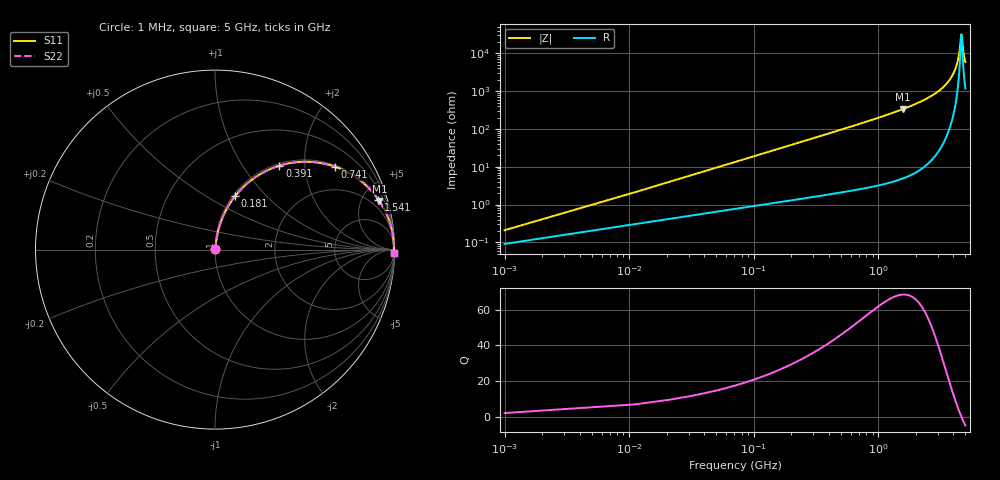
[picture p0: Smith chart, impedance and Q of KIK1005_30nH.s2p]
!version-3
!date-01.2023
!Series
# MHz S RI R 50
!Freq ReS11 ImS11 ReS21 ImS21 ReS12 ImS12 ReS22 ImS22
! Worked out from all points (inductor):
!   501 points, 1 MHz to 5 GHz, reference 50 ohm
!   read as one part in series: L = 30 nH near 21 MHz
!   highest Q = 68.5 at 1.581 GHz (marker M1), where L = 33.9 nH
!   self-resonance near 4.641 GHz
!   S11 on the Smith chart (normalised r, x): 1 MHz: 1.00, +0.00; 181 MHz: 1.02, +0.68; 391 MHz: 1.04, +1.48; 741 MHz: 1.05, +2.87; 1.541 GHz: 1.10, +6.53; 5 GHz: open
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1  0.00091 0.00188  0.9991 -0.00188  0.9991 -0.00188  0.00091 0.00188
31  0.00838 0.0577  0.9916 -0.0577  0.9916 -0.0577  0.00838 0.0577
51  0.0154 0.0941  0.9846 -0.0941  0.9846 -0.0941  0.0154 0.0941
101  0.0431 0.1806  0.9569 -0.1806  0.9569 -0.1806  0.0431 0.1806
181  0.1131 0.2994  0.8869 -0.2994  0.8869 -0.2994  0.1131 0.2994
271  0.215 0.3964  0.785 -0.3964  0.785 -0.3964  0.215 0.3964
391  0.3587 0.4675  0.6413 -0.4675  0.6413 -0.4675  0.3587 0.4675
741  0.6697 0.4613  0.3303 -0.4613  0.3303 -0.4613  0.6697 0.4613
841  0.7253 0.4378  0.2747 -0.4378  0.2747 -0.4378  0.7253 0.4378
1141  0.8359 0.3627  0.1641 -0.3627  0.1641 -0.3627  0.8359 0.3627
1541  0.9108 0.2778  0.0892 -0.2778  0.0892 -0.2778  0.9108 0.2778
1581  0.9158 0.2705  0.0842 -0.2705  0.0842 -0.2705  0.9158 0.2705
1671  0.9258 0.2548  0.0742 -0.2548  0.0742 -0.2548  0.9258 0.2548
2501  0.9753 0.1465  0.0247 -0.1465  0.0247 -0.1465  0.9753 0.1465
3341  0.9917 0.0758  0.00833 -0.0758  0.00833 -0.0758  0.9917 0.0758
3831  0.9954 0.044  0.00461 -0.044  0.00461 -0.044  0.9954 0.044
4171  0.9966 0.0245  0.00343 -0.0245  0.00343 -0.0245  0.9966 0.0245
4421  0.9969 0.0113  0.00311 -0.0113  0.00311 -0.0113  0.9969 0.0113
4641  0.9969 0.000237  0.00314 -0.000237  0.00314 -0.000237  0.9969 0.000237
4681  0.9968 -0.00171  0.00317 0.00171  0.00317 0.00171  0.9968 -0.00171
4841  0.9966 -0.00933  0.00338 0.00933  0.00338 0.00933  0.9966 -0.00933
5000  0.9963 -0.0167  0.00371 0.0167  0.00371 0.0167  0.9963 -0.0167
